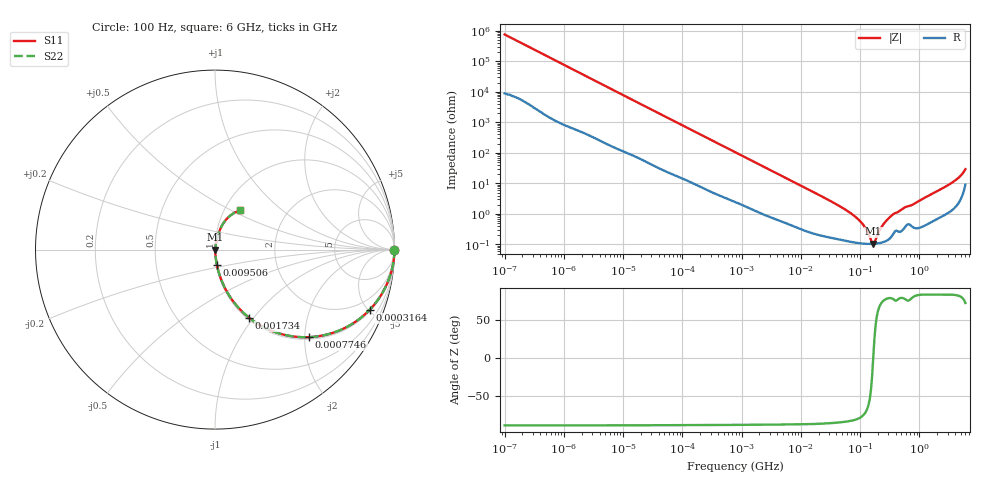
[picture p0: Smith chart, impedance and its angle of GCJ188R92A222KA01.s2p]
!Murata Part Number: GCJ188R92A222KA01
!These Parameters are Measured in Series Mode Connection
!Data Generated on Mar 13, 2026
!  o--ll--o
!Port1  Port2
!  o------o
!Operation Temp=25[degC], DC Bias Voltage=0[V]
!Freq. Start=100[Hz] Stop=6[GHz] 401[Steps]
# Hz S RI R 50
!Freq.(Hz) S11(Real) S11(Imag) S21(Real) S21(Imag) S12(Real) S12(Imag) S22(Real) S22(Imag)
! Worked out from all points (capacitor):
!   401 points, 100 Hz to 6 GHz, reference 50 ohm
!   read as one part in series: C = 2.12 nF near 109 Hz
!   lowest |Z| = 105 mohm at 166.9 MHz (marker M1)
!   series resonance near 167.1 MHz, so ESL is about 430 pH
!   S11 on the Smith chart (normalised r, x): 100 Hz: open; 316.4 kHz: 1.10, -5.09; 774.6 kHz: 1.05, -2.10; 1.734 MHz: 1.02, -0.95; 9.506 MHz: 1.01, -0.18; 6 GHz: 1.18, +0.56
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100  1 -0.000134  1.6e-06 0.000134  1.6e-06 0.000134  1 -0.000134
2008  1 -0.00262  3.96e-05 0.00262  3.96e-05 0.00262  1 -0.00262
40335  0.9966 -0.051  0.00343 0.051  0.00343 0.051  0.9966 -0.051
118133  0.9759 -0.1444  0.0241 0.1444  0.0241 0.1444  0.9759 -0.1444
316350  0.8614 -0.3356  0.1386 0.3356  0.1386 0.3356  0.8614 -0.3356
774597  0.5248 -0.4877  0.4752 0.4877  0.4752 0.4877  0.5248 -0.4877
1734173  0.1908 -0.3802  0.8092 0.3802  0.8092 0.3802  0.1908 -0.3802
3394479  0.0628 -0.2283  0.9372 0.2283  0.9372 0.2283  0.0628 -0.2283
9506416  0.0111 -0.0878  0.9889 0.0878  0.9889 0.0878  0.0111 -0.0878
1.555665e7  0.00528 -0.0541  0.9947 0.0541  0.9947 0.0541  0.00528 -0.0541
4.556224e7  0.00175 -0.0177  0.9982 0.0177  0.9982 0.0177  0.00175 -0.0177
8.154455e7  0.00122 -0.00827  0.9988 0.00827  0.9988 0.00827  0.00122 -0.00827
1.166697e8  0.00108 -0.00392  0.9989 0.00392  0.9989 0.00392  0.00108 -0.00392
1.526266e8  0.00104 -0.000973  0.999 0.000973  0.999 0.000973  0.00104 -0.000973
1.669249e8  0.00105 -1.02e-05  0.999 1.02e-05  0.999 1.02e-05  0.00105 -1.02e-05
1.825626e8  0.00106 0.000957  0.9989 -0.000957  0.9989 -0.000957  0.00106 0.000957
2.388273e8  0.00119 0.00397  0.9988 -0.00397  0.9988 -0.00397  0.00119 0.00397
3.124326e8  0.00158 0.00741  0.9984 -0.00741  0.9984 -0.00741  0.00158 0.00741
5.59173e8  0.00369 0.0155  0.9963 -0.0155  0.9963 -0.0155  0.00369 0.0155
7.650043e8  0.00415 0.0194  0.9958 -0.0194  0.9958 -0.0194  0.00415 0.0194
3.205649e9  0.0193 0.089  0.9807 -0.089  0.9807 -0.089  0.0193 0.089
6e9  0.1394 0.2194  0.8606 -0.2194  0.8606 -0.2194  0.1394 0.2194
